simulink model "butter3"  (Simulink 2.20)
settings: Solver=VariableStepDiscrete  StartTime=0.0  StopTime=20.0  RelTol=1e-3  AbsTol=1e-6
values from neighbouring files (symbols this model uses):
  a = input('Inserisci il dato da graficare [1=PIDNL 2=PD 3=PID]: ')    [grp.m]    (also in grp1.m = input('Inserisci il dato da graficare [1..3]'))
undefined symbols (not defined in the file or in its folder): b, NL

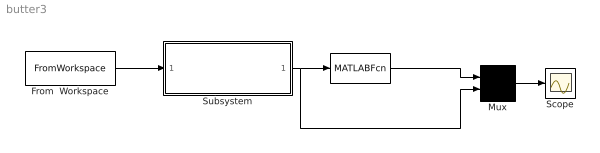
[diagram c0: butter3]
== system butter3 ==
  " " : MATLABFcn  MATLABFcn=NL(u(1))  OutputWidth=-1
  From  Workspace : FromWorkspace  VariableName=[out(:,1),out(:,12)]
  Mux : Mux  Inputs=2
  Scope : Scope
  Subsystem : Subsystem  mask(Filtro di Butterworth){ordine=3, freq=0.6/16}
      mask prompts: ordine "Ordine del filtro"; freq "Parametro K per ricavare la Freq. di taglio Ft"
      mask help: Attenzione! Considerare il parametro Fc come la frequanza di campionamento del segnale di ingresso, per cui la frequanza di taglio diviene Ft=K*Fc;
      mask init:
      | [b,a]=butter(ordine,freq);
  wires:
  " "/1 -> Mux/1
  From  Workspace/1 -> Subsystem/1(In1)
  Subsystem/1(Out1) -> " "/1, Mux/2
  Mux/1 -> Scope/1

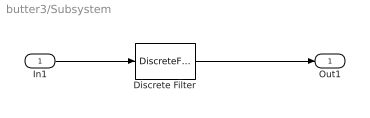
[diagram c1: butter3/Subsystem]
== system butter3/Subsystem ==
  In1 : Inport  Port=1  PortWidth=-1  SampleTime=-1
  Discrete Filter : DiscreteFilter  Numerator=b  Denominator=a  SampleTime=.033
  Out1 : Outport  Port=1
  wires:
  In1/1 -> Discrete Filter/1
  Discrete Filter/1 -> Out1/1
